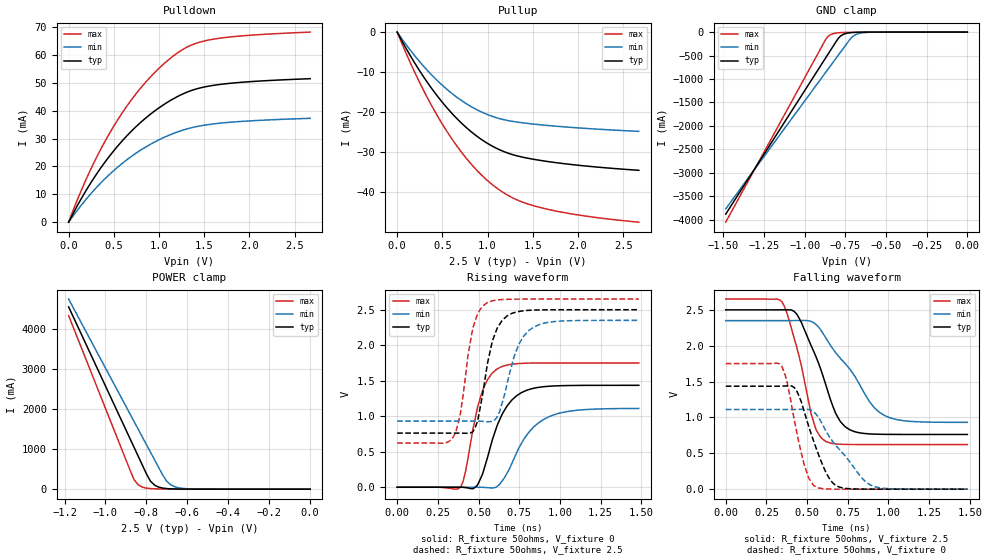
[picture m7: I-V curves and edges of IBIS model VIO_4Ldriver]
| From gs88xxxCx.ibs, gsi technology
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|  signals   DQA1-DQA9, DQB1-DQB9, DQC1-DQC9, DQD1-DQD9
[Model]   VIO_4Ldriver
Model_type   I/O
Polarity   Non-Inverting
Vinl  =   0.54v
Vinh  =   1.10v
Vmeas =   0.90v
Cref  =   0pF
Rref  =   50
Vref  =   0.90v
|  variable   typ   min   max
C_comp   3.0pF   2.5pF   3.5pF
|  variable   typ   min   max
[Temperature Range]   50   0   100
|  variable   typ   min   max
[Voltage Range]   2.5   2.35   2.65
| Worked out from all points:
|   slope of the pulldown table from 0 to 0.375 V, typ, clamps not added: 18.5 ohm
|   slope of the pullup table from 0 to 0.375 V, typ, clamps not added: 27 ohm
|   GND clamp passes 1 mA (typ) near -0.61 V on its own axis
|   POWER clamp passes 1 mA (typ) near -0.59 V on its own axis
|   rising waveform, R_fixture 50ohms, V_fixture 0: 20-80 % time 139ps typ, 178ps min, 102ps max; typ from 0 V to 1.44 V
|   rising waveform, R_fixture 50ohms, V_fixture 2.5: 20-80 % time 91ps typ, 113ps min, 77.9ps max; typ from 0.763 V to 2.5 V
|   falling waveform, R_fixture 50ohms, V_fixture 2.5: 20-80 % time 170ps typ, 258ps min, 125ps max; typ from 2.5 V to 0.763 V
|   falling waveform, R_fixture 50ohms, V_fixture 0: 20-80 % time 132ps typ, 216ps min, 95.9ps max; typ from 1.44 V to 0 V
[Pulldown]
| voltage   typ   min   max
0V        -364.2pA   -1.049nA   -219.7pA
108mV     6.602mA    4.763mA    8.908mA
243mV     13.97mA    10.09mA    18.82mA
378mV     20.45mA    14.78mA    27.52mA
513mV     26.13mA    18.89mA    35.13mA
648mV     31.07mA    22.46mA    41.77mA
810mV     36.14mA    26.09mA    48.59mA
1.134V    43.78mA    31.48mA    58.96mA
1.35V     47.11mA    33.78mA    63.37mA
1.566V    48.86mA    35.08mA    65.4mA
1.971V    50.29mA    36.25mA    66.92mA
2.673V    51.44mA    37.24mA    68.14mA
[Pullup]
| voltage (VDDQ-Vout)   typ   min   max
0V        284.9pA    1.042nA    119pA
243mV     -9.504mA   -7.26mA    -12.37mA
378mV     -14mA      -10.65mA   -18.28mA
513mV     -17.95mA   -13.59mA   -23.53mA
648mV     -21.37mA   -16.1mA    -28.13mA
783mV     -24.27mA   -18.18mA   -32.1mA
918mV     -26.66mA   -19.85mA   -35.45mA
1.053V    -28.56mA   -21.1mA    -38.2mA
1.296V    -30.81mA   -22.43mA   -41.71mA
1.566V    -32.07mA   -23.17mA   -43.83mA
2.025V    -33.39mA   -24.03mA   -45.87mA
2.673V    -34.61mA   -24.86mA   -47.6mA
[GND Clamp]
| voltage   typ   min   max
-1.485V   -3.884A    -3.771A    -4.056A
-885mV    -626.9mA   -926.9mA   -247.2mA
-870mV    -545.6mA   -856mA     -153.5mA
-855mV    -464.4mA   -785mA     -89.11mA
-825mV    -301.9mA   -643.2mA   -32.88mA
-795mV    -141.5mA   -501.4mA   -15.38mA
-780mV    -86.61mA   -430.5mA   -11.65mA
-750mV    -32.85mA   -288.8mA   -7.734mA
-705mV    -8.727mA   -95.28mA   -4.834mA
-660mV    -2.907mA   -24.97mA   -2.925mA
-555mV    -316.7uA   -1.176mA   -484.9uA
0V        -354.4pA   -1.034nA   -211.5pA
[POWER Clamp]
| voltage (VDDQ-Vout)   typ   min   max
-1.18V    4.545A     4.74A      4.328A
-880mV    1.258A     1.875A     474.1mA
-860mV    1.039A     1.684A     234.3mA
-840mV    820.4mA    1.493A     107.4mA
-820mV    601.5mA    1.302A     50.64mA
-780mV    197.3mA    920.5mA    14.28mA
-760mV    99.71mA    729.7mA    9.034mA
-720mV    26.23mA    348.2mA    4.898mA
-700mV    13.96mA    192.6mA    3.916mA
-660mV    4.495mA    57.55mA    2.579mA
-560mV    510.5uA    2.941mA    648.3uA
0V        285pA      1.042nA    119.1pA
[Ramp]
| voltage   typ   min   max
dV/dt_r   0.46/174p   0.27/249p   0.72/134p
dV/dt_f   0.47/176p   0.32/258p   0.64/129p
R_load  =   50ohms
[Rising Waveform]
C_fixture =   0.0pF
R_fixture =   50ohms
V_fixture =   0
| Time   V(typ)   V(min)   V(max)
0s        4.324nV    15.83nV    2.057nV
390ps     300.6uV    336.9uV    3.926mV
420ps     -4.922mV   614.7uV    220.6mV
480ps     -880.9uV   799.1uV    973.5mV
525ps     186.7mV    -711.2uV   1.362V
630ps     950.5mV    42.86mV    1.684V
735ps     1.29V      488.1mV    1.74V
810ps     1.376V     776.9mV    1.748V
900ps     1.415V     954.8mV    1.75V
1.485ns   1.435V     1.11V      1.751V
[Rising Waveform]
C_fixture =   0.0pF
R_fixture =   50ohms
V_fixture =   2.5
V_fixture_min =  2.35
V_fixture_max =  2.65
| Time   V(typ)   V(min)   V(max)
0s        762.5mV    931mV      621.9mV
345ps     762.3mV    931mV      709.4mV
390ps     761.7mV    931.3mV    1.056V
435ps     760.3mV    931.7mV    1.854V
480ps     843.4mV    931mV      2.348V
555ps     1.743V     921.8mV    2.601V
645ps     2.349V     1.185V     2.644V
750ps     2.476V     2.023V     2.649V
840ps     2.495V     2.256V     2.65V
1.485ns   2.5V       2.35V      2.65V
[Falling Waveform]
C_fixture =   0.0pF
R_fixture =   50ohms
V_fixture =   2.5
V_fixture_min =  2.35
V_fixture_max =  2.65
| Time   V(typ)   V(min)   V(max)
0s        2.5V       2.35V      2.65V
345ps     2.5V       2.35V      2.615V
435ps     2.446V     2.351V     1.991V
540ps     1.925V     2.322V     938.8mV
615ps     1.456V     2.109V     664.4mV
675ps     1.061V     1.904V     630.7mV
735ps     869mV      1.749V     624mV
885ps     770.3mV    1.215V     622.1mV
975ps     764.4mV    1.028V     622mV
1.485ns   762.7mV    931.5mV    622mV
[Falling Waveform]
C_fixture =   0.0pF
R_fixture =   50ohms
V_fixture =   0
| Time   V(typ)   V(min)   V(max)
0s        1.435V     1.111V     1.751V
345ps     1.436V     1.111V     1.715V
375ps     1.44V      1.11V      1.519V
435ps     1.377V     1.112V     811.3mV
510ps     877mV      1.11V      154.9mV
555ps     575.7mV    1.046V     33.25mV
615ps     237.1mV    814.3mV    4.086mV
675ps     52.88mV    613.1mV    593.3uV
885ps     328.4uV    62.21mV    9.486uV
1.485ns   1.109uV    5.329uV    458.8nV
